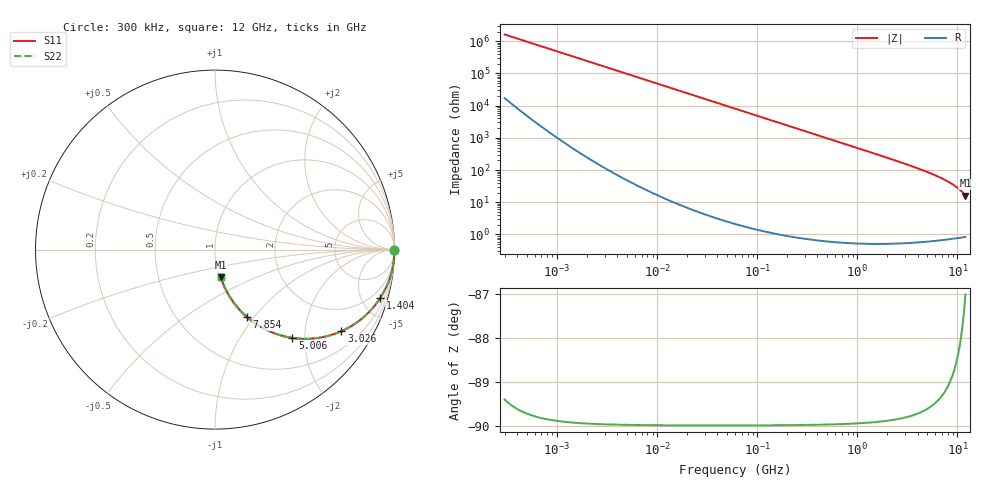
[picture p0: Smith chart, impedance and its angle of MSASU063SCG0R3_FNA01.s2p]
! MSASU063SCG0R3_FNA01  S-PARAMETER MODEL  ( Standard Model )
! Model Generated by TAIYO YUDEN Corporation (http://www.ty-top.com)
! Version 1.0
! TAIYO YUDEN Control No. 240819
! Copyright(c) 2024 TAIYO YUDEN CO.,LTD. All Rights Reserved.
! Product Description (link to TY-COMPAS)
! https://ds.yuden.co.jp/TYCOMPAS/or/detail?pn=MSASU063SCG0R3CFNA01&u=M
! Products Name : Multilayer Ceramic Capacitors
! Characteristics :
!  Capacitance : 0.3 [pF] , Rated Voltage : 50 [V] , TCC : CG / C0G
!  Case Size : 0.6 x 0.3 / 0.024 x 0.012 [mm/inch] , Thickness : 0.3 / 0.012 [mm/inch]
!  (Conditions: Temperature = 25 [degC] , DC Bias Voltage = 0 [V])
! External Node Assignments :
!  1  o---| |---o  2
! GND o---------o GND
! Frequency Range : 0.3MHz  -  12000MHz  [ 401 STEP ]
# MHZ S RI R 50
! Freq[MHz].  S11 Real  S11 Imag  S21 Real  S21 Imag  S12 Real  S12 Imag  S22 Real  S22 Imag
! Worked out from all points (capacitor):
!   401 points, 300 kHz to 12 GHz, reference 50 ohm
!   read as one part in series: C = 327 fF near 316.3 kHz
!   lowest |Z| = 16 ohm at 12 GHz (marker M1)
!   S11 on the Smith chart (normalised r, x): 300 kHz: open; 1.404 GHz: 1.01, -6.87; 3.026 GHz: 1.01, -3.09; 5.006 GHz: 1.01, -1.74; 7.854 GHz: 1.01, -0.92; 12 GHz: 1.02, -0.32
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0.3  1 -6.17e-05  6.54e-07 6.17e-05  6.54e-07 6.17e-05  1 -6.17e-05
0.458357  1 -9.43e-05  5.38e-07 9.43e-05  5.38e-07 9.43e-05  1 -9.43e-05
0.496271  1 -0.000102  5.23e-07 0.000102  5.23e-07 0.000102  1 -0.000102
1.769972  1 -0.000364  5.44e-07 0.000364  5.44e-07 0.000364  1 -0.000364
10.44266  1 -0.00215  5.34e-06 0.00215  5.34e-06 0.00215  1 -0.00215
60  0.9998 -0.0123  0.000156 0.0123  0.000156 0.0123  0.9998 -0.0123
164.1901  0.9988 -0.0337  0.00115 0.0337  0.00115 0.0337  0.9988 -0.0337
353.9943  0.9947 -0.0725  0.00532 0.0725  0.00532 0.0725  0.9947 -0.0725
743.2595  0.9769 -0.1497  0.0231 0.1497  0.0231 0.1497  0.9769 -0.1497
1048.836  0.9549 -0.207  0.0451 0.207  0.0451 0.207  0.9549 -0.207
1403.667  0.9215 -0.2682  0.0785 0.2682  0.0785 0.2682  0.9215 -0.2682
2088.533  0.8387 -0.3667  0.1613 0.3667  0.1613 0.3667  0.8387 -0.3667
2514.07  0.7792 -0.4134  0.2208 0.4134  0.2208 0.4134  0.7792 -0.4134
3026.31  0.7039 -0.4548  0.2961 0.4548  0.2961 0.4548  0.7039 -0.4548
3944.255  0.5698 -0.4927  0.4302 0.4927  0.4302 0.4927  0.5698 -0.4927
5006.236  0.4304 -0.4917  0.5696 0.4917  0.5696 0.4917  0.4304 -0.4917
6188.031  0.3044 -0.4554  0.6956 0.4554  0.6956 0.4554  0.3044 -0.4554
7854.144  0.1772 -0.3743  0.8228 0.3743  0.8228 0.3743  0.1772 -0.3743
8732.115  0.1297 -0.3265  0.8703 0.3265  0.8703 0.3265  0.1297 -0.3265
9708.23  0.0893 -0.2729  0.9107 0.2729  0.9107 0.2729  0.0893 -0.2729
10511.28  0.0641 -0.2296  0.9359 0.2296  0.9359 0.2296  0.0641 -0.2296
12000  0.0325 -0.1531  0.9675 0.1531  0.9675 0.1531  0.0325 -0.1531
